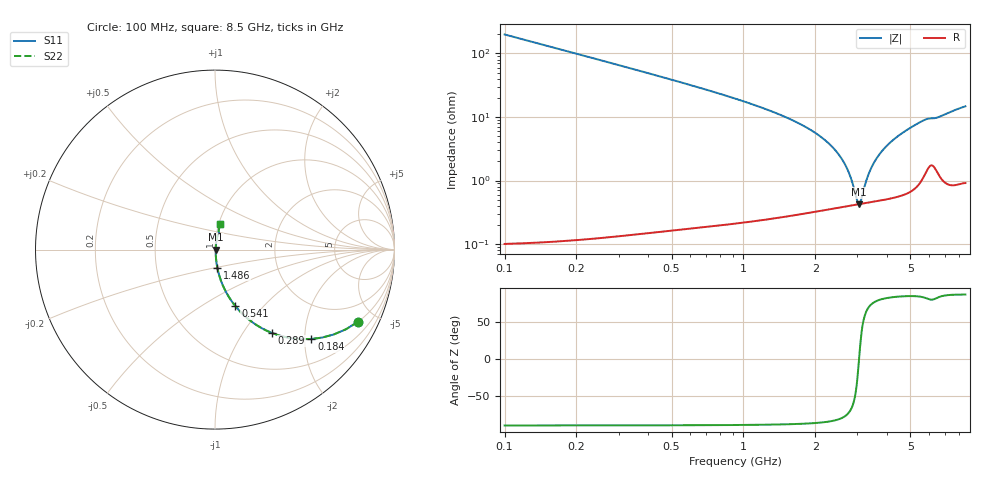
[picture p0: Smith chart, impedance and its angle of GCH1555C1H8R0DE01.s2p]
!Murata Part Number: GCH1555C1H8R0DE01
!These Parameters are Measured in Series Mode Connection
!Data Generated on Jun 19, 2026
!  o--ll--o
!Port1  Port2
!  o------o
!Operation Temp=25[degC], DC Bias Voltage=0[V]
!Freq. Start=100[MHz] Stop=9[GHz] 401[Steps]
# Hz S RI R 50
!Freq.(Hz) S11(Real) S11(Imag) S21(Real) S21(Imag) S12(Real) S12(Imag) S22(Real) S22(Imag)
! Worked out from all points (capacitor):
!   401 points, 100 MHz to 8.5 GHz, reference 50 ohm
!   read as one part in series: C = 8 pF near 142 MHz
!   lowest |Z| = 426 mohm at 3.04 GHz (marker M1)
!   series resonance near 3.05 GHz, so ESL is about 340 pH
!   S11 on the Smith chart (normalised r, x): 100 MHz: 1.00, -3.97; 184 MHz: 1.00, -2.15; 289 MHz: 1.00, -1.36; 541 MHz: 1.00, -0.71; 1.486 GHz: 1.01, -0.20; 8.5 GHz: 1.02, +0.29
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1e8  0.7978 -0.4014  0.2022 0.4014  0.2022 0.4014  0.7978 -0.4014
1.84e8  0.5369 -0.4981  0.4631 0.4981  0.4631 0.4981  0.5369 -0.4981
2.89e8  0.3175 -0.4646  0.6825 0.4646  0.6825 0.4646  0.3175 -0.4646
3.94e8  0.198 -0.397  0.802 0.397  0.802 0.397  0.198 -0.397
5.41e8  0.1133 -0.3146  0.8867 0.3146  0.8867 0.3146  0.1133 -0.3146
9.19e8  0.0389 -0.188  0.9611 0.188  0.9611 0.188  0.0389 -0.188
1.486e9  0.0128 -0.0998  0.9872 0.0998  0.9872 0.0998  0.0128 -0.0998
1.507e9  0.0123 -0.0976  0.9877 0.0976  0.9877 0.0976  0.0123 -0.0976
2.074e9  0.00587 -0.0506  0.9941 0.0506  0.9941 0.0506  0.00587 -0.0506
2.452e9  0.00447 -0.0281  0.9955 0.0281  0.9955 0.0281  0.00447 -0.0281
2.725e9  0.00414 -0.0144  0.9959 0.0144  0.9959 0.0144  0.00414 -0.0144
2.914e9  0.00414 -0.00582  0.9959 0.00582  0.9959 0.00582  0.00414 -0.00582
2.998e9  0.00418 -0.00219  0.9958 0.00219  0.9958 0.00219  0.00418 -0.00219
3.04e9  0.00422 -0.000411  0.9958 0.000411  0.9958 0.000411  0.00422 -0.000411
3.103e9  0.00428 0.00221  0.9957 -0.00221  0.9957 -0.00221  0.00428 0.00221
3.334e9  0.0046 0.0114  0.9954 -0.0114  0.9954 -0.0114  0.0046 0.0114
3.523e9  0.00498 0.0185  0.995 -0.0185  0.995 -0.0185  0.00498 0.0185
3.859e9  0.00586 0.0303  0.9941 -0.0303  0.9941 -0.0303  0.00586 0.0303
4.3e9  0.00739 0.0448  0.9926 -0.0448  0.9926 -0.0448  0.00739 0.0448
5.707e9  0.0191 0.0859  0.9809 -0.0859  0.9809 -0.0859  0.0191 0.0859
7.114e9  0.0212 0.1102  0.9788 -0.1102  0.9788 -0.1102  0.0212 0.1102
8.5e9  0.0296 0.1413  0.9704 -0.1413  0.9704 -0.1413  0.0296 0.1413
